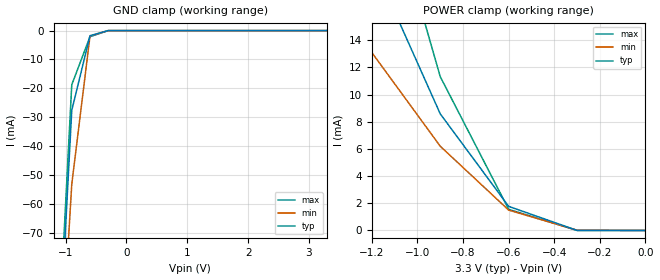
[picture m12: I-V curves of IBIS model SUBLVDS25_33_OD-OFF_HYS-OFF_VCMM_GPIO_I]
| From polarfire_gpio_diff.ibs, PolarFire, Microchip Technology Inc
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|   SUBLVDS25_33_OD-OFF_HYS-OFF_VCMM_GPIO_I
[Model]   SUBLVDS25_33_OD-OFF_HYS-OFF_VCMM_GPIO_I
Model_type  Input
Vinl =   0.775
Vinh =   1.025
|   typ   min   max
C_comp_pullup   2.605e-12   2.605e-12   2.76e-12
C_comp_pulldown  2.605e-12   2.605e-12   2.76e-12
[Temperature Range]  25C   100C   -40C
[Voltage Range]  3.3V   3.15V   3.45V
[GND_clamp]
|Voltage   I(typ)   I(min)   I(max)
-3.3V     -1.138A    -1.018A    -1.313A
-1.2V     -147.1mA   -159mA     -141.3mA
-900mV    -27.64mA   -53.3mA    -18.77mA
-600mV    -1.775mA   -1.87mA    -2.115mA
-300mV    -1.462uA   -4.313uA   -854.3nA
3.3V      1.341uA    1.798uA    1.108uA
[POWER_clamp]
|Voltage   I(typ)   I(min)   I(max)
-3.3V     238mA      182.9mA    319.1mA
-3V       189mA      142.2mA    262.9mA
-2.7V     150.7mA    108.6mA    215.8mA
-2.4V     116.7mA    82.12mA    171.9mA
-2.1V     85.28mA    59.16mA    128.7mA
-1.8V     55.36mA    38.84mA    85.19mA
-1.5V     34.04mA    23.18mA    52.5mA
-1.2V     19.85mA    13.1mA     28.9mA
-900mV    8.583mA    6.201mA    11.32mA
-600mV    1.775mA    1.5mA      1.556mA
-300mV    6.226uA    20.37uA    3.158uA
0V        0A         0A         0A
